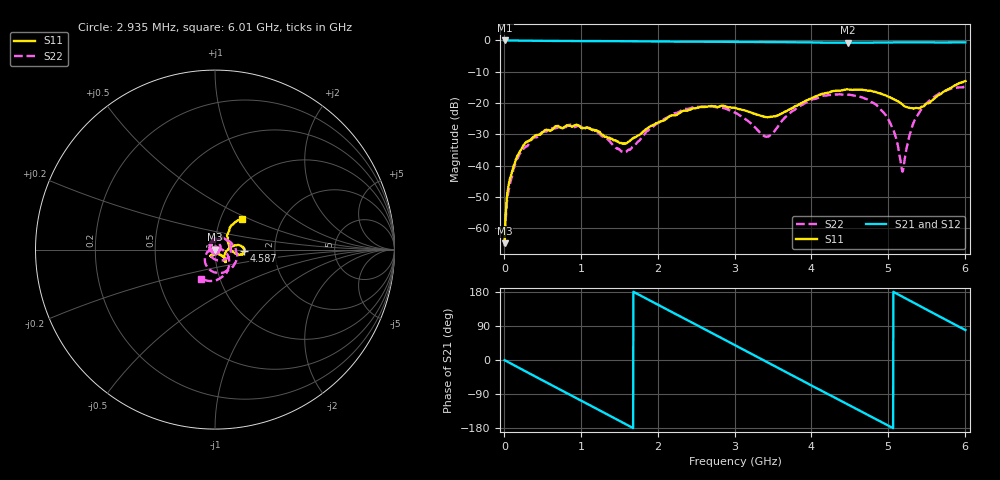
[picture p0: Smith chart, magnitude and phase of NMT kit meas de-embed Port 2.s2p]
! Carlisle Launcher - Use on Port1  07/02/2020  12:31:25
! Ref Plane: 0.000 mm
# MHZ S MA R  50
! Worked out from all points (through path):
!   2048 points, 2.935 MHz to 6.01 GHz, reference 50 ohm
!   highest |S21| = 0.00 dB at 8.804 MHz (marker M1); lowest = -0.7 dB at 4.478 GHz (marker M2)
!   group delay of S21, straight-line fit = 296 ps
!   lowest |S11| = -64.7 dB at 2.935 MHz (marker M3), VSWR 1.00, Z = 50.1 - j0.0245 ohm
!   |S11| at or under -10 dB: start of sweep to end of sweep
!   |S22| runs from -65.7 to -14.8 dB; largest |S21 - S12| = 0.0063
!   S11 on the Smith chart (normalised r, x): 2.935 MHz: 1.00, -0.00; 4.587 GHz: 1.39, -0.03; 6.01 GHz: 1.26, +0.45
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2.9346  0.00058 -24.9  0.9995 -0.4  0.9994 -0.3  0.00052 -37.6
8.8037  0.00103 -52.8  0.9995 -1.0  0.9992 -1.0  0.00086 -58.3
44.0186  0.004 -70.3  0.998 -4.9  0.9981 -4.9  0.00343 -94.8
79.2334  0.00658 -73.9  0.997 -8.7  0.9971 -8.8  0.00548 -103.6
161.4014  0.01366 -90.1  0.9948 -17.6  0.9948 -17.7  0.01267 -114.9
264.1113  0.02243 -95.3  0.9919 -28.7  0.9918 -28.7  0.01941 -141.0
648.54  0.04053 -120.0  0.9834 -69.8  0.983 -69.9  0.03993 150.1
1006.558  0.03994 -123.2  0.9773 -107.9  0.9771 -107.9  0.04155 75.9
1567.06  0.02273 -79.7  0.9721 -167.8  0.9722 -167.8  0.0167 -98.0
2007.246  0.04953 -42.5  0.963 145.3  0.9631 145.3  0.04838 121.8
2511.992  0.08399 -45.7  0.9542 91.8  0.9548 91.7  0.08742 27.0
3007.934  0.08378 -49.6  0.9478 38.9  0.9486 38.8  0.07015 -61.8
3427.578  0.0596 -26.0  0.9421 -5.8  0.9423 -5.9  0.02915 166.6
4008.623  0.1202 11.2  0.9297 -67.8  0.932 -67.9  0.1139 5.0
4478.154  0.165 0.7  0.918 -117.3  0.9209 -117.2  0.1359 -67.5
4586.733  0.1635 -3.4  0.9199 -128.8  0.9208 -128.7  0.1293 -83.8
5009.311  0.126 -10.9  0.9291 -173.5  0.9298 -173.5  0.05375 -154.8
5191.254  0.09426 -4.3  0.931 166.8  0.9335 166.8  0.00802 92.0
5320.375  0.08275 12.9  0.9328 153.0  0.936 152.9  0.04391 -2.4
5461.235  0.08868 36.3  0.933 137.7  0.9369 137.6  0.08737 -29.8
5728.281  0.1528 56.0  0.9295 109.0  0.9337 108.8  0.1536 -72.4
6009.999  0.2247 48.8  0.9309 79.0  0.9335 78.8  0.1818 -114.7
